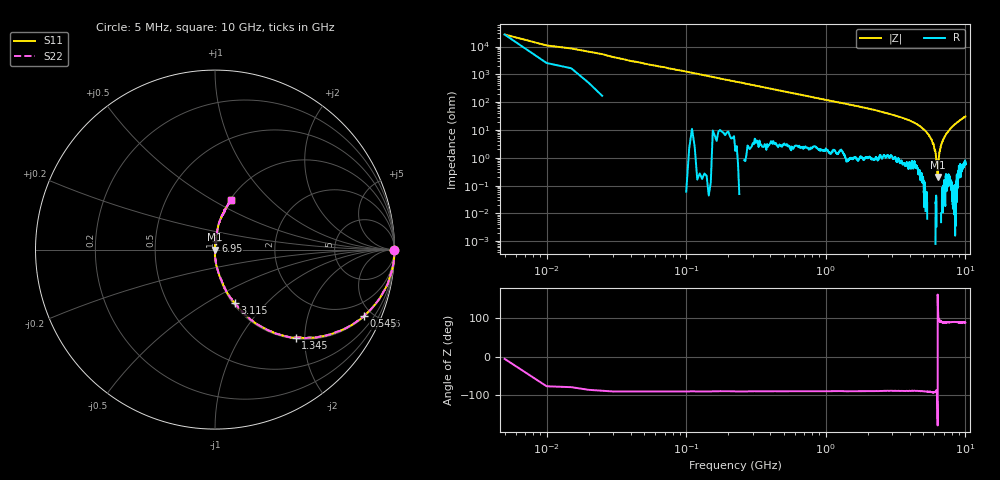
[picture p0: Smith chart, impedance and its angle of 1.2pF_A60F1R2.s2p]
! Amotech Co.,Ltd.
! http://www.amotech.co.kr/
! Part Number: A60F1R2
! These Parameters are Measured in Series Mode Connection
! Operation Temp=25[degC], DC Bias Voltage=0[V]
! Freq. Start=5[MHz] Stop=10[GHz], 2000[Steps]
! Date: Monday, July 20, 2020, 03:12:51
# GHZ S RI R 50.000000
!Freq.(Hz) S11(Real) S11(Imag) S21(Real) S21(Imag) S12(Real) S12(Imag) S22(Real) S22(Imag)
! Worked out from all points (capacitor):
!   2000 points, 5 MHz to 10 GHz, reference 50 ohm
!   read as one part in series: C = 1.27 pF near 55 MHz
!   lowest |Z| = 206 mohm at 6.315 GHz (marker M1)
!   series resonance near 6.325 GHz, so ESL is about 500 pH
!   S11 on the Smith chart (normalised r, x): 5 MHz: open; 545 MHz: 1.05, -4.49; 1.345 GHz: 1.03, -1.81; 3.115 GHz: 1.02, -0.67; 6.95 GHz: 1.00, +0.09; 10 GHz: 1.01, +0.61
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0.005  0.9964 -0.00035  0.00363 0.00035  0.00363 0.00035  0.9964 -0.00035
0.075  0.9963 -0.0609  0.00373 0.0609  0.00373 0.0609  0.9963 -0.0609
0.15  0.9859 -0.1177  0.0141 0.1177  0.0141 0.1177  0.9859 -0.1177
0.31  0.9385 -0.2341  0.0615 0.2341  0.0615 0.2341  0.9385 -0.2341
0.545  0.8318 -0.3685  0.1682 0.3685  0.1682 0.3685  0.8318 -0.3685
1.345  0.4503 -0.4902  0.5497 0.4902  0.5497 0.4902  0.4503 -0.4902
1.675  0.345 -0.4695  0.655 0.4695  0.655 0.4695  0.345 -0.4695
3.115  0.1088 -0.2967  0.8912 0.2967  0.8912 0.2967  0.1088 -0.2967
3.34  0.0895 -0.2704  0.9105 0.2704  0.9105 0.2704  0.0895 -0.2704
5.005  0.013 -0.1064  0.987 0.1064  0.987 0.1064  0.013 -0.1064
5.53  0.00262 -0.0604  0.9974 0.0604  0.9974 0.0604  0.00262 -0.0604
5.91  -0.000224 -0.0321  1 0.0321  1 0.0321  -0.000224 -0.0321
6.11  0.000305 -0.016  0.9997 0.016  0.9997 0.016  0.000305 -0.016
6.23  -0.000358 -0.00755  1 0.00755  1 0.00755  -0.000358 -0.00755
6.315  -0.00193 -0.000745  1.002 0.000745  1.002 0.000745  -0.00193 -0.000745
6.345  -0.00264 0.00234  1.003 -0.00234  1.003 -0.00234  -0.00264 0.00234
6.5  -0.00137 0.014  1.001 -0.014  1.001 -0.014  -0.00137 0.014
6.67  0.000368 0.0264  0.9996 -0.0264  0.9996 -0.0264  0.000368 0.0264
6.95  0.00285 0.0466  0.9971 -0.0466  0.9971 -0.0466  0.00285 0.0466
7.515  0.00897 0.0879  0.991 -0.0879  0.991 -0.0879  0.00897 0.0879
8.335  0.0239 0.1523  0.9761 -0.1523  0.9761 -0.1523  0.0239 0.1523
10  0.0915 0.2768  0.9085 -0.2768  0.9085 -0.2768  0.0915 0.2768
